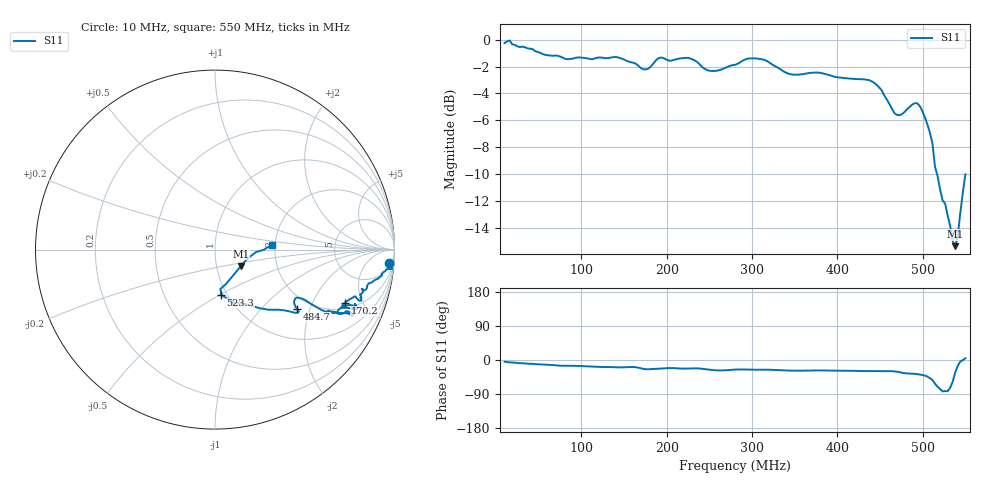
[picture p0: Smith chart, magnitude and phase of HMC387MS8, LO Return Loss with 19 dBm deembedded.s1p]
!Hittite Microwave Corporation
!12 Elizabeth Drive
!Chelmsford, MA 01824
!Tel: 978-250-3343
!Fax: 978-250-3373
!Device: HMC387MS8, 450-500 MHz, GaAs MMIC High IP3 Mixer in 8-lead plastic SMT package
!Misc: LO Return Loss with 19 dBm, Room
# MHZ S MA R 50
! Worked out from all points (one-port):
!   183 points, 10 MHz to 550 MHz, reference 50 ohm
!   lowest |S11| = -15.3 dB at 538.1 MHz (marker M1), VSWR 1.41, Z = 65.6 - j12.3 ohm
!   |S11| at or under -10 dB: 516.8 MHz to end of sweep
!   S11 on the Smith chart (normalised r, x): 10 MHz: 9, -23; 170.2 MHz: 2.37, -3.61; 484.7 MHz: 1.70, -1.63; 523.3 MHz: 0.94, -0.50; 550 MHz: 1.92, +0.11
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10  0.971 -4.3
15.934  0.993 -6.2
27.802  0.938 -8.4
78.242  0.857 -15.1
146.484  0.852 -19.5
161.319  0.82 -18.6
170.22  0.782 -22.2
179.121  0.783 -24.5
193.956  0.858 -22.4
214.725  0.851 -22.4
232.527  0.838 -22.1
256.264  0.765 -27.2
280  0.806 -25.2
312.637  0.844 -25.6
348.242  0.741 -28.1
416.484  0.716 -28.4
443.187  0.691 -29.5
466.923  0.533 -30.1
484.725  0.563 -35.7
493.626  0.58 -37.2
502.527  0.514 -41.2
511.429  0.411 -52.6
514.396  0.337 -62.6
523.297  0.253 -82.7
529.231  0.222 -82.4
538.132  0.171 -32.1
541.099  0.187 -15.9
550  0.316 4.6
